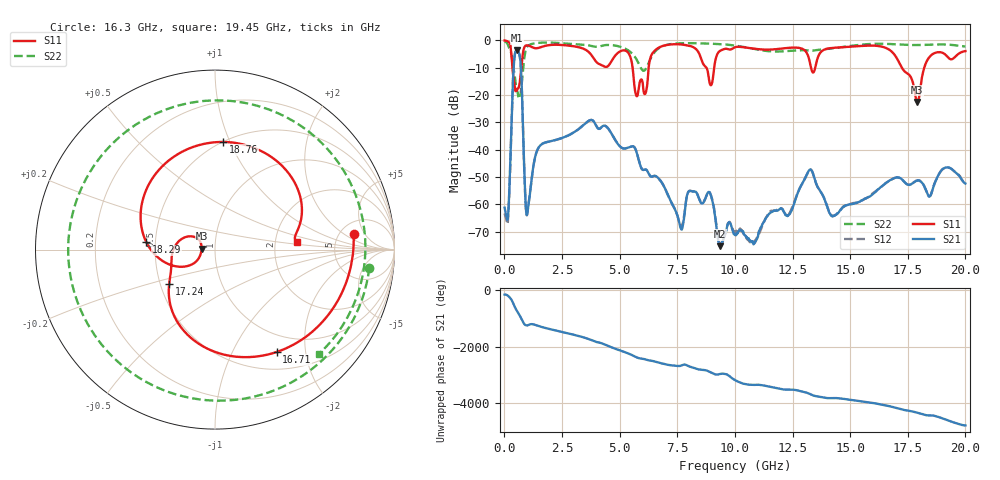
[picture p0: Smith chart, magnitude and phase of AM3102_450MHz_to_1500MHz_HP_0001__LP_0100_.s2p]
!Agilent Technologies,E8364B,MY43040894,A.07.50.67
!Agilent E8364B: A.07.50.67
!Date: Thursday, January 11, 2018 05:20:29
!Correction: S11(Full 2 Port(1,2))
!S21(Full 2 Port(1,2))
!S12(Full 2 Port(1,2))
!S22(Full 2 Port(1,2))
!S2P File: Measurements: S11, S21, S12, S22:
# Hz S  dB  R 50
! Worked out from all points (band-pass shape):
!   1601 points, 10 MHz to 20 GHz, reference 50 ohm
!   highest |S21| = -3.66 dB at 534.7 MHz (marker M1); lowest = -75.2 dB at 9.355 GHz (marker M2)
!   |S21| within 3 dB of the highest: 432.9 MHz to 682.2 MHz (249.3 MHz wide, 44.7 % of centre)
!   lowest |S11| = -22.5 dB at 17.91 GHz (marker M3), VSWR 1.16, Z = 43 + j0.427 ohm
!   |S11| at or under -10 dB: 348.6 MHz to 736.6 MHz (388 MHz wide, 71.5 % of centre); 5.562 GHz to 6.259 GHz (696.1 MHz wide, 11.8 % of centre); 17.24 GHz to 18.22 GHz (972.4 MHz wide, 5.48 % of centre)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
!   |S22| runs from -21.3 to -0.4 dB; largest |S21 - S12| = 0.0031
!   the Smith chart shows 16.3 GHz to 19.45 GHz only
!   S11 on the Smith chart (normalised r, x): 16.3 GHz: 6.61, +2.98; 16.71 GHz: 0.73, -1.51; 17.24 GHz: 0.56, -0.24; 18.29 GHz: 0.45, +0.04; 18.76 GHz: 0.50, +0.95; 19.45 GHz: 2.66, +0.27
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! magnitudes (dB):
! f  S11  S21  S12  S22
! 10 MHz  -0.1  -61.2  -63.3  -0.4
! 534.7 MHz  -18.4  -3.7  -3.7  -18.3
! 997 MHz  -1.8  -63.2  -63.2  -2.3
! 1.509 GHz  -2.7  -38.9  -38.9  -0.9
! 3.346 GHz  -2.8  -31.6  -31.6  -1.6
! 5.745 GHz  -20.4  -41.1  -41.1  -7.2
! 6.682 GHz  -2.8  -50.4  -50.4  -3.0
! 7.669 GHz  -1.5  -69.0  -68.1  -1.1
! 8.906 GHz  -15.6  -55.6  -55.5  -1.2
! 9.355 GHz  -3.9  -75.2  -74.2  -1.4
! 10.01 GHz  -2.5  -71.2  -69.9  -1.9
! 13.34 GHz  -11.2  -47.7  -47.7  -3.8
! 14.24 GHz  -2.8  -64.4  -64.2  -2.9
! 16.3 GHz  -2.2  -53.8  -53.9  -1.3
! 16.68 GHz  -3.3  -51.4  -51.4  -1.3
! 16.71 GHz  -3.5  -51.2  -51.2  -1.3
! 17.24 GHz  -9.9  -50.7  -50.8  -1.6
! 17.91 GHz  -22.5  -51.3  -51.2  -1.7
! 18.29 GHz  -8.3  -54.6  -54.8  -1.7
! 18.76 GHz  -4.4  -50.3  -50.4  -1.5
! 19.45 GHz  -6.8  -47.4  -47.4  -1.7
! 20 GHz  -4.0  -52.3  -52.3  -2.3
